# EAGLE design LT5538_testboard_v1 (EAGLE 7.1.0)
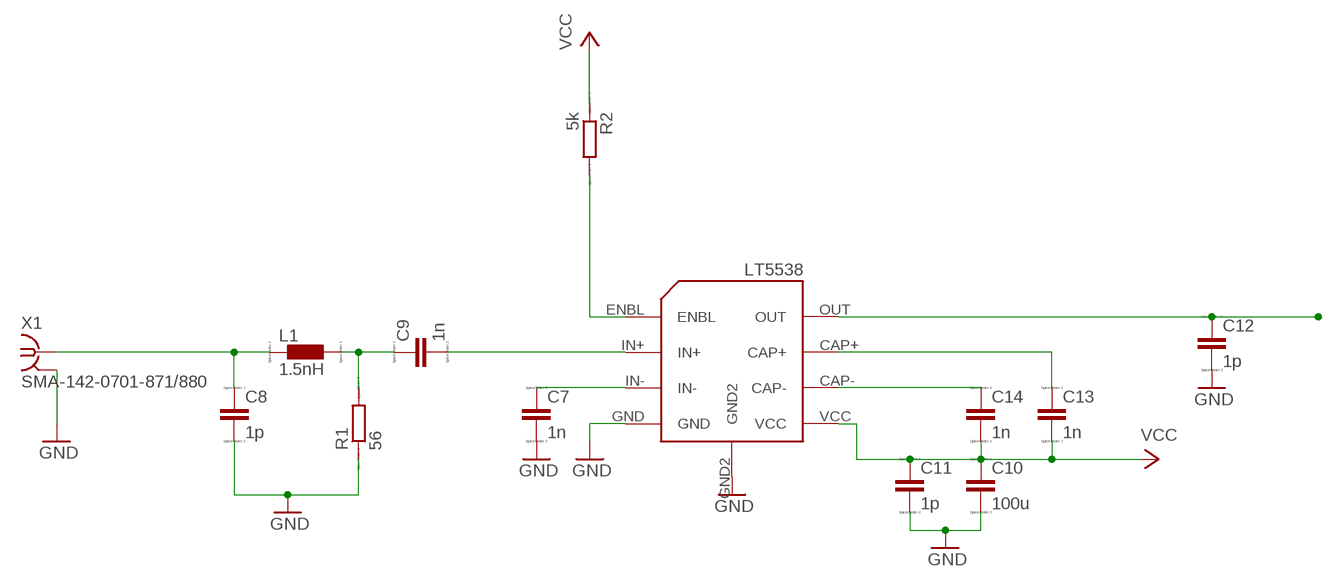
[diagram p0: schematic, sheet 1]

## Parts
C7  1n  C  [C0805]
C8  1p  C  [C0805]
C9  1n  C  [C0805]
C10  100u  C  [C0805]
C11  1p  C  [C0805]
C12  1p  C  [C0805]
C13  1n  C  [C0805]
C14  1n  C  [C0805]
L1  1.5nH  L  [L1812]
R1  56  R  [R0805]
R2  5k  R  [R0805]
U$1  LT5538  [LT5538]
X1  SMA-142-0701-871/880  [SMA-142-0701-871]

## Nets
GND: C7.2 C8.2 C10.2 C11.2 C12.2 R1.1 U$1.GND U$1.GND2 X1.2@1 X1.2@2 X1.2@3 X1.2@4
N$1: C7.1 U$1.IN-
N$2: C9.2 U$1.IN+
N$3: C9.1 L1.1 R1.2
N$4: C8.1 L1.2 X1.1
N$5: C14.1 U$1.CAP-
N$6: R2.2 U$1.ENBL
N$7: C12.1 U$1.OUT
N$8: C13.1 U$1.CAP+
VCC: C10.1 C11.1 C13.2 C14.2 R2.1 U$1.VCC

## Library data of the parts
C7-C9 C11-C14 = eagle-ltspice:C: CAPACITOR, European symbol; SPICEMODEL: 1p; SPICEPREFIX: C
C10 = eagle-ltspice:C: CAPACITOR, European symbol; SPICEMODEL: NONE; SPICEPREFIX: C
L1 = eagle-ltspice:L: INDUCTOR, European symbol; SPICEMODEL: NONE; SPICEPREFIX: L
R1 R2 = eagle-ltspice:R: RESISTOR, European symbol; SPICEMODEL: NONE; SPICEPREFIX: R
U$1 = LT5538:LT5538
X1 = con-coax:SMA-: SMA 50 Ohm End Launch Jack Receptacle - Round Contact; MF: JOHNSON COMPONENTS; MPN: 142-0701-871; OC_FARNELL: 1339835; OC_NEWARK: 91B6105

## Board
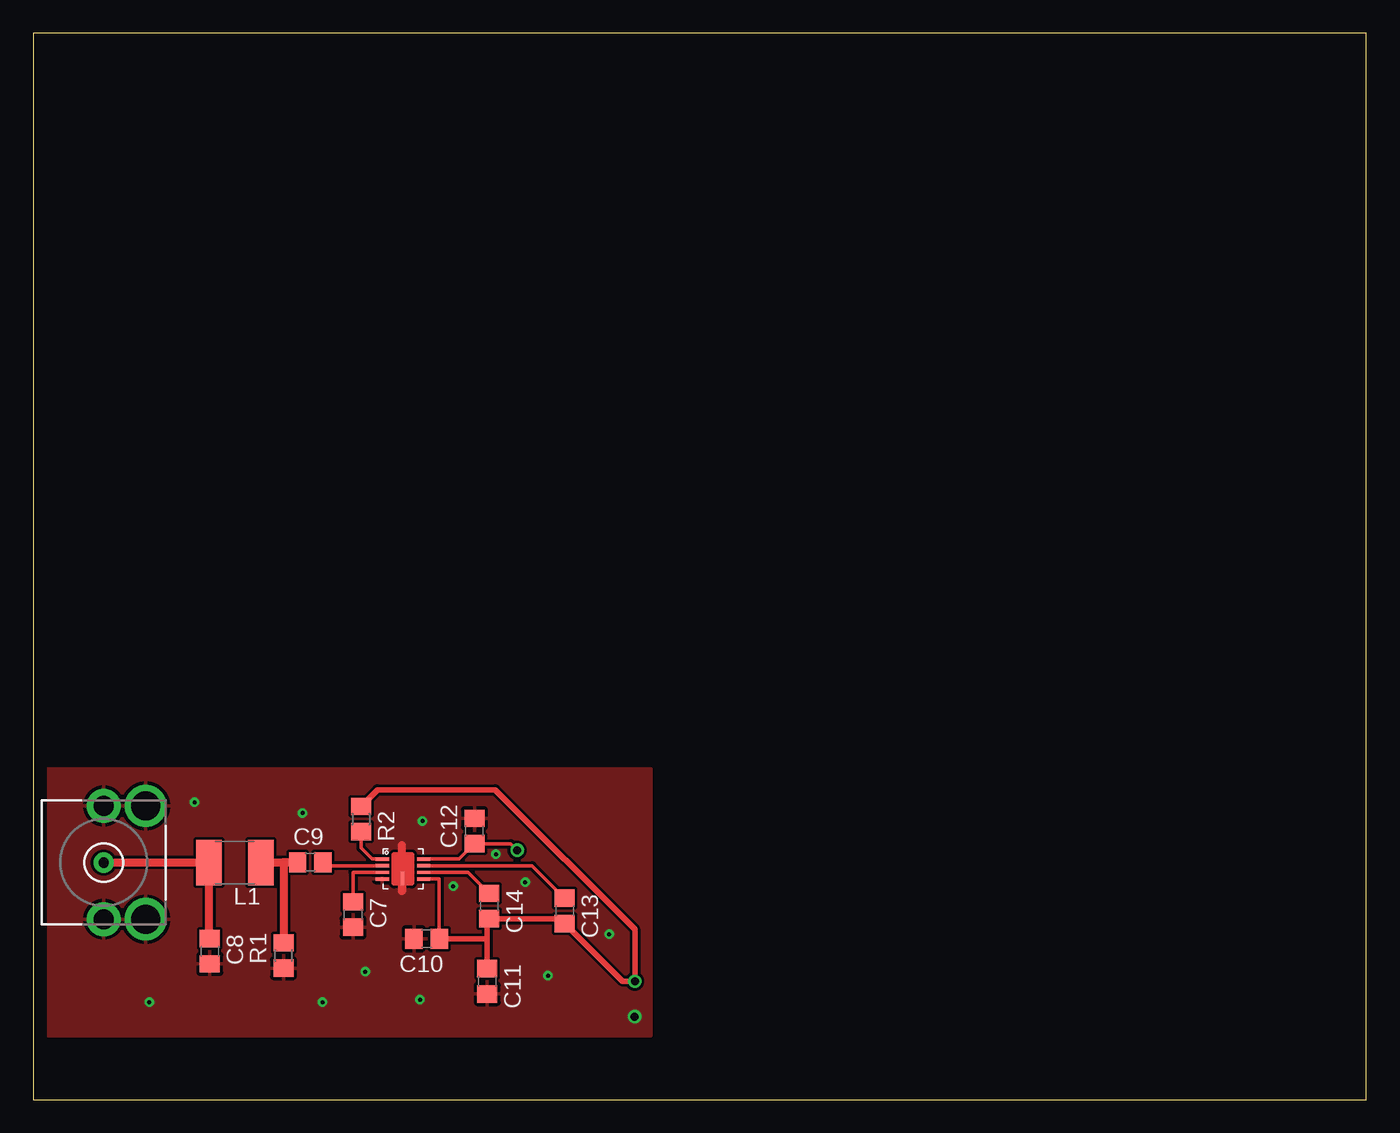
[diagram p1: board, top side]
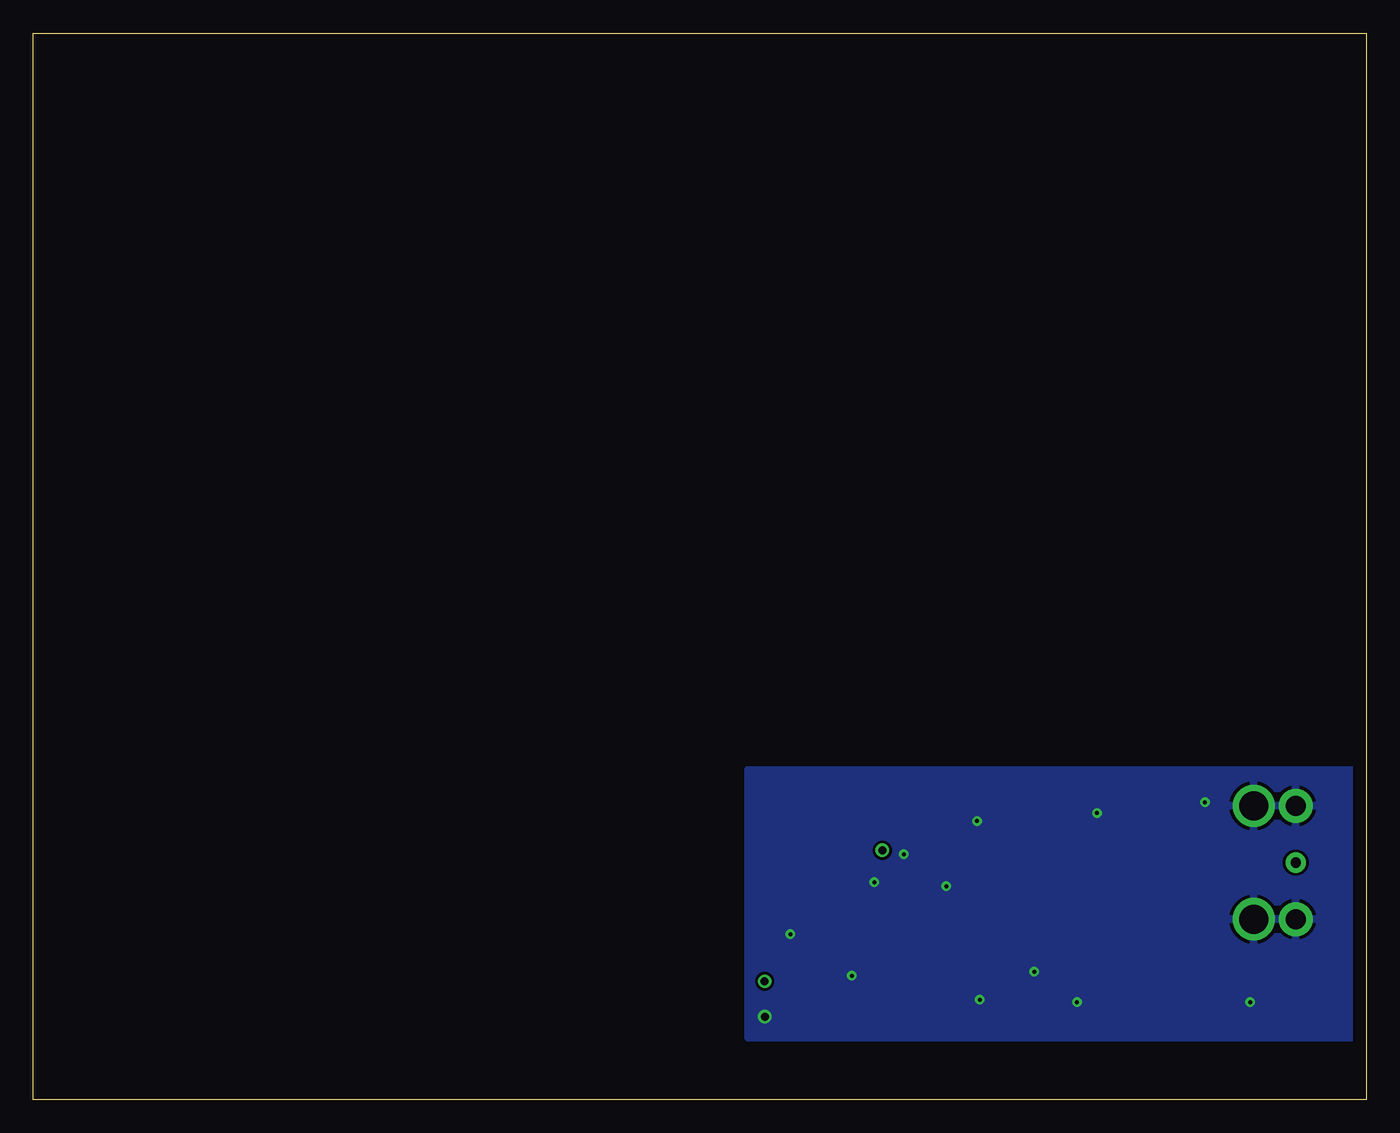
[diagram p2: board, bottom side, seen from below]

Size 100 x 80 mm. Coordinates in mm from the lower left corner, seen from the top.
Outline: 0,0 100,0 100,80 0,80 0,0
Copper layers (1*16): Top 0.035mm / dielectric 1.5mm / Bottom 0.035mm
Design rules "default": minimum track width 10mil, minimum drill 24mil, track to track 8mil, track to pad 8mil, pad to pad 8mil, via to via 8mil, smd to smd 8mil, copper to edge 40mil, drill to drill 8mil, minimum pad ring 10mil, minimum via ring 8mil, stop-mask expansion 4mil, vias tented up to drill 0mil, thermal gap 10mil

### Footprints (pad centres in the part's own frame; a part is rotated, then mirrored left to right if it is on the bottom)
C0805 = smd 1.3 x 1.5: 1 -0.95,0; 2 0.95,0
L1812 = smd 1.9 x 3.4: 1 -1.95,0; 2 1.95,0
R0805 = smd 1.3 x 1.5: 1 -0.95,0; 2 0.95,0
LT5538 = smd 0.25 x 1: CAP+ -0.22,1.58; CAP- 0.28,1.58; ENBL -0.72,-1.52; GND 0.78,-1.52; IN+ -0.22,-1.52; IN- 0.28,-1.52; OUT -0.72,1.58; VCC 0.78,1.58 | smd 1 x 0.25: GND2 0.73,-0.02
SMA-142-0701-871 = drill 0.762 pad 1.524: 1 0,0 | drill 1.524 pad 2.54: 2@1 -4.255,0; 2@2 4.255,0 | drill 2.159 pad 2.794: 2@3 -4.255,-3.15; 2@4 4.255,-3.15

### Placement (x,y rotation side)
C7  23.99,13.88 270 top
C8  13.24,11.13 270 top
C9  20.78,17.8 0 top
C10  29.5,12.07 180 top
C11  34.06,8.87 270 top
C12  33.1,20.14 90 top
C13  39.87,14.16 270 top
C14  34.21,14.52 270 top
L1  15.13,17.78 180 top
R1  18.78,10.81 90 top
R2  24.58,21.05 270 top
U$1  27.7,17.33 270 top
X1  5.28,17.78 90 top

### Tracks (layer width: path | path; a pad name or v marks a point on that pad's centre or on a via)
GND  (via drill 0.3 pad 0.3, 0.6)
  Top 0.61: U$1.GND2 27.68,15.68 27.65,15.65 27.65,19.1
  other vias: 45.11,6.22 12.1,22.3 20.2,21.5 29.2,20.9 36.9,16.3 31.5,16 24.9,9.6 43.2,12.4 29,7.5 38.6,9.3 21.7,7.3 8.7,7.3 34.7,18.4
  pour Top: 0,24.8 46.35,24.8 46.35,4.8 0,4.8
  pour Bottom: 0.05,4.65 46.35,4.65 46.35,24.75 0.05,24.75
N$1
  Top 0.254: U$1.IN- 23.99,17.05 C7.1
N$2
  Top 0.254: U$1.IN+ 21.98,17.55 arc-90 C9.2
N$3
  Top 0.61: L1.1 17.1,17.8 C9.1 18.78,17.8 R1.2
N$4
  Top 0.61: X1.1 L1.2 13.18,12.08 C8.1
N$5
  Top 0.254: U$1.CAP- 32.63,17.05 C14.1
N$6
  Top 0.254: U$1.ENBL 25.4,18.05 24.58,18.87 R2.2
N$7  (via drill 0.6)
  Top 0.254: U$1.OUT 31.96,18.05 C12.1 35.81,19.19 v36.3,18.7
N$8
  Top 0.254: U$1.CAP+ 37.43,17.55 C13.1
VCC  (via drill 0.6)
  Top 0.254: U$1.VCC 30.45,16.55 C10.1
  Top 0.406: C10.1 34.06,12.07 | 34.06,12.07 C11.1 | 34.06,12.07 34.06,13.57 C14.2 39.87,13.57 C13.2 44.21,8.87 v45.13,8.87 45.13,12.77 34.65,23.25 25.83,23.25 R2.1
